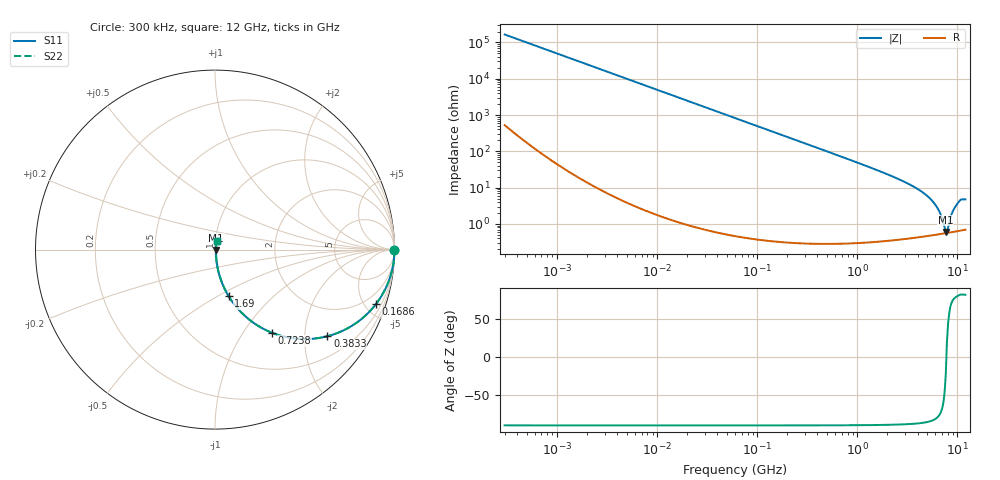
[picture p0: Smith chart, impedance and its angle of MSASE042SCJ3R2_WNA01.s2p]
! MSASE042SCJ3R2_WNA01  S-PARAMETER MODEL  ( General Type )
! Model Generated by TAIYO YUDEN Corporation (http://www.ty-top.com)
! Version 1.0
! TAIYO YUDEN Control No. 120810
! Copyright(c) 2012 TAIYO YUDEN CO.,LTD. All Rights Reserved.
! Product Description (link to TY-COMPAS)
! https://ds.yuden.co.jp/TYCOMPAS/or/detail?pn=MSASE042SCJ3R2BWNA01&u=M
! Products Name : Multilayer Ceramic Capacitors
! Characteristics :
!  Capacitance : 3.2 pF , Rated Voltage : 16V , TCC : CJ / C0J
!  Case Size : 0.4 x 0.2 / 0.016 x 0.008 [mm/inch] , Thickness : 0.2 / 0.008 [mm/inch]
!  (Conditions: Temperature = 25 degC , DC Bias Current/Voltage = 0A / 0V)
! External Node Assignments :
!  1  o---| |---o  2
! GND o---------o GND
! Frequency Range : 0.3MHz  -  12000MHz  [ 401 STEP ]
# MHz S RI R 50
! Freq[MHz].  S11 Real  S11 Imag  S21 Real  S21 Imag  S12 Real  S12 Imag  S22 Real  S22 Imag
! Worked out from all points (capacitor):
!   401 points, 300 kHz to 12 GHz, reference 50 ohm
!   read as one part in series: C = 3.2 pF near 316.3 kHz
!   lowest |Z| = 599 mohm at 7.649 GHz (marker M1)
!   series resonance near 7.755 GHz, so ESL is about 130 pH
!   S11 on the Smith chart (normalised r, x): 300 kHz: open; 168.6 MHz: 1.01, -5.90; 383.3 MHz: 1.01, -2.59; 723.8 MHz: 1.01, -1.36; 1.69 GHz: 1.01, -0.56; 12 GHz: 1.01, +0.09
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0.3  1 -0.000603  2.27e-06 0.000603  2.27e-06 0.000603  1 -0.000603
1.769972  1 -0.00356  1.48e-05 0.00356  1.48e-05 0.00356  1 -0.00356
10.44266  0.9996 -0.021  0.000447 0.021  0.000447 0.021  0.9996 -0.021
60  0.9856 -0.1188  0.0144 0.1188  0.0144 0.1188  0.9856 -0.1188
168.5979  0.8968 -0.3037  0.1032 0.3037  0.1032 0.3037  0.8968 -0.3037
353.9943  0.6629 -0.4717  0.3371 0.4717  0.3371 0.4717  0.6629 -0.4717
383.2761  0.6264 -0.4827  0.3736 0.4827  0.3736 0.4827  0.6264 -0.4827
723.8279  0.3181 -0.4636  0.6819 0.4636  0.6819 0.4636  0.3181 -0.4636
1105.905  0.1645 -0.3674  0.8355 0.3674  0.8355 0.3674  0.1645 -0.3674
1689.663  0.0756 -0.2587  0.9244 0.2587  0.9244 0.2587  0.0756 -0.2587
2088.533  0.0496 -0.2095  0.9504 0.2095  0.9504 0.2095  0.0496 -0.2095
3642.919  0.0152 -0.1047  0.9848 0.1047  0.9848 0.1047  0.0152 -0.1047
5140.631  0.00758 -0.0539  0.9924 0.0539  0.9924 0.0539  0.00758 -0.0539
6354.153  0.00576 -0.0258  0.9942 0.0258  0.9942 0.0258  0.00576 -0.0258
6879.757  0.00551 -0.0157  0.9945 0.0157  0.9945 0.0157  0.00551 -0.0157
7448.838  0.00549 -0.00553  0.9945 0.00553  0.9945 0.00553  0.00549 -0.00553
7648.807  0.00553 -0.00222  0.9945 0.00222  0.9945 0.00222  0.00553 -0.00222
8064.993  0.00569 0.00543  0.9943 -0.00543  0.9943 -0.00543  0.00569 0.00543
8966.534  0.00639 0.021  0.9936 -0.021  0.9936 -0.021  0.00639 0.021
9708.23  0.00717 0.0313  0.9928 -0.0313  0.9928 -0.0313  0.00717 0.0313
10793.46  0.0086 0.0456  0.9914 -0.0456  0.9914 -0.0456  0.0086 0.0456
12000  0.00901 0.0461  0.991 -0.0461  0.991 -0.0461  0.00901 0.0461
